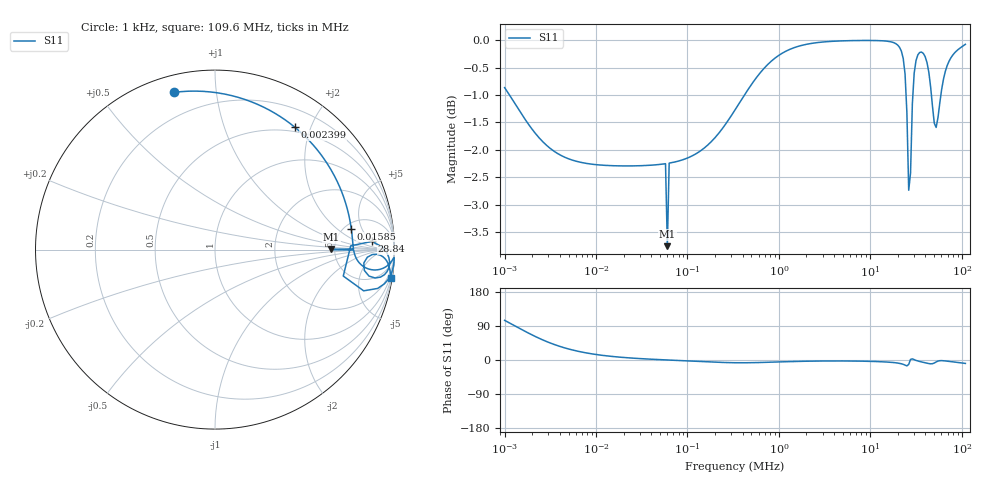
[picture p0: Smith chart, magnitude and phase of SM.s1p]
! EM Consulting and Software
! Touchstone file was created on 2026-03-05  19:00:35
# HZ S RI R 50.0000
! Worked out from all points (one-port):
!   253 points, 1 kHz to 109.6 MHz, reference 50 ohm
!   lowest |S11| = -3.8 dB at 60.26 kHz (marker M1), VSWR 4.69, Z = 235 + j0.741 ohm
!   |S11| at or under -10 dB: nowhere
!   S11 on the Smith chart (normalised r, x): 1 kHz: 0.08, +0.77; 2.399 kHz: 0.43, +1.76; 15.85 kHz: 5.71, +3.27; 28.84 MHz: 13, +5; 109.6 MHz: 1, -13
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1000  -0.229 0.8759
1513.561  0.13 0.848
2398.833  0.4434 0.6828
4365.158  0.6555 0.4288
7943.282  0.7324 0.2436
15848.93  0.7591 0.1174
18197.01  0.7614 0.1
57543.99  0.7715 0.00343
60255.96  0.6487 0.000915
63095.73  0.7724 -0.00256
79432.82  0.7755 -0.0175
331131.1  0.8569 -0.1084
1445440  0.9818 -0.068
6025596  0.9982 -0.0467
1.380384e7  0.9954 -0.0835
2.089296e7  0.9734 -0.1522
2.398833e7  0.9062 -0.2164
2.511886e7  0.8282 -0.2297
2.630268e7  0.7146 -0.1473
2.754229e7  0.7561 0.0209
2.884032e7  0.8744 0.0459
3.311311e7  0.9689 -0.0447
4.365158e7  0.9224 -0.1532
5.011872e7  0.8318 -0.1158
5.495409e7  0.8488 -0.0424
6.025596e7  0.9011 -0.0258
7.585776e7  0.9608 -0.0706
1.096478e8  0.9793 -0.1559
